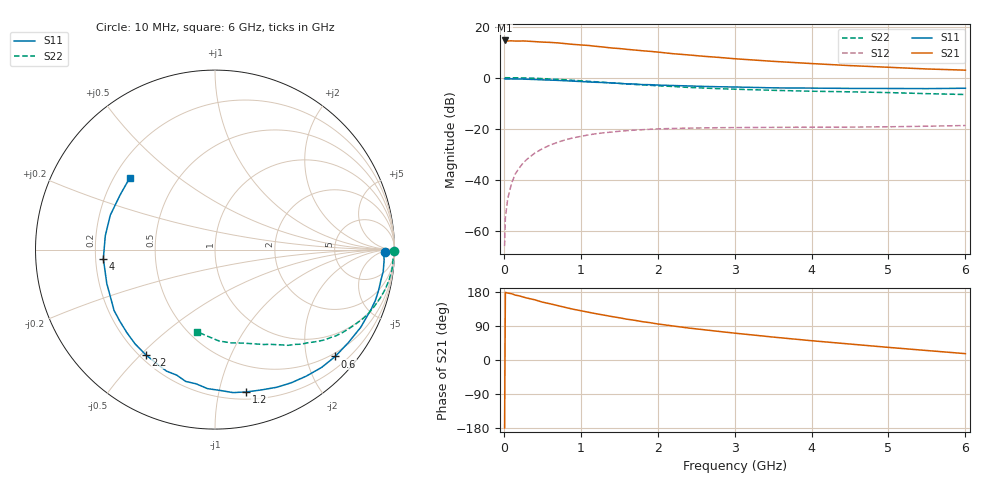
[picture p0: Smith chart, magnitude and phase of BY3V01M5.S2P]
! SIEMENS Small Signal Semiconductors
! BFY420
! Si NPN RF SIEGET Grounded Emitter Transistor in MICRO-X
! VCE = 3 V  IC = 1.5 mA
! Common Emitter S-Parameters:  October  1996
# GHz  S  MA  R  50
!  f  S11  S21  S12  S22
! GHz  MAG  ANG  MAG  ANG  MAG  ANG  MAG  ANG
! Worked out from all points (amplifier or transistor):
!   36 points, 10 MHz to 6 GHz, reference 50 ohm
!   highest |S21| = 14.6 dB at 10 MHz (marker M1)
!   |S21| within 3 dB of that: start of sweep to 1.425 GHz
!   unconditionally stable (mu >= 1): 4.266 GHz to end of sweep
!   at 250 MHz: K = 0.05, MSG = 23.9 dB, |S12| = -33.5 dB
!   at 1.4 GHz: K = 0.24, MSG = 16.5 dB, |S12| = -21.3 dB
!   at 6 GHz: K = 1.28, MAG = 7.7 dB, |S12| = -18.7 dB
!   S11 on the Smith chart (normalised r, x): 10 MHz: 35, -8; 600 MHz: 0.43, -2.57; 1.2 GHz: 0.26, -1.21; 2.2 GHz: 0.22, -0.52; 4 GHz: 0.23, -0.04; 6 GHz: 0.26, +0.34
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0.01  0.9466 -0.7  5.357 -179.5  0.0005 100.2  0.9995 -0.3
0.02  0.9396 -1.6  5.333 178.6  0.0018 83.7  0.9982 -0.6
0.05  0.9441 -3.4  5.239 176.7  0.0042 87.1  0.997 -1.7
0.1  0.9451 -7.4  5.265 175.0  0.0085 85.5  0.993 -3.4
0.15  0.9399 -10.5  5.22 171.2  0.0131 82.7  0.9935 -5.2
0.2  0.9393 -14.0  5.212 169.3  0.017 81.1  0.9921 -6.6
0.3  0.9312 -20.9  5.196 163.5  0.0252 77.5  0.9844 -10.0
0.5  0.9061 -34.8  4.977 152.8  0.0405 70.2  0.9588 -16.4
0.6  0.8962 -41.6  4.91 148.4  0.0477 66.0  0.9431 -19.5
0.8  0.8693 -54.2  4.647 138.7  0.0606 58.5  0.907 -25.4
1.1  0.8225 -72.1  4.273 126.1  0.0756 49.1  0.8485 -32.9
1.2  0.8117 -77.7  4.111 122.1  0.0798 46.3  0.8293 -35.3
1.6  0.7551 -98.0  3.587 107.7  0.0916 36.5  0.7526 -43.2
2  0.7164 -116.0  3.17 95.1  0.0992 28.9  0.6931 -49.6
2.2  0.7017 -123.3  2.948 89.8  0.1012 25.7  0.6713 -52.6
2.4  0.6887 -130.3  2.789 84.4  0.1026 23.2  0.6445 -55.4
2.8  0.6634 -143.2  2.491 75.3  0.1047 18.8  0.6074 -60.3
3.5  0.6317 -162.7  2.089 60.5  0.1064 13.8  0.5653 -68.1
4  0.6242 -175.4  1.89 50.9  0.1069 11.7  0.5423 -73.8
4.5  0.616 172.8  1.723 42.1  0.1075 10.0  0.5279 -80.0
5.5  0.6101 150.2  1.48 25.0  0.1119 9.5  0.486 -94.4
6  0.6204 140.1  1.403 16.8  0.1155 9.5  0.4679 -102.5
